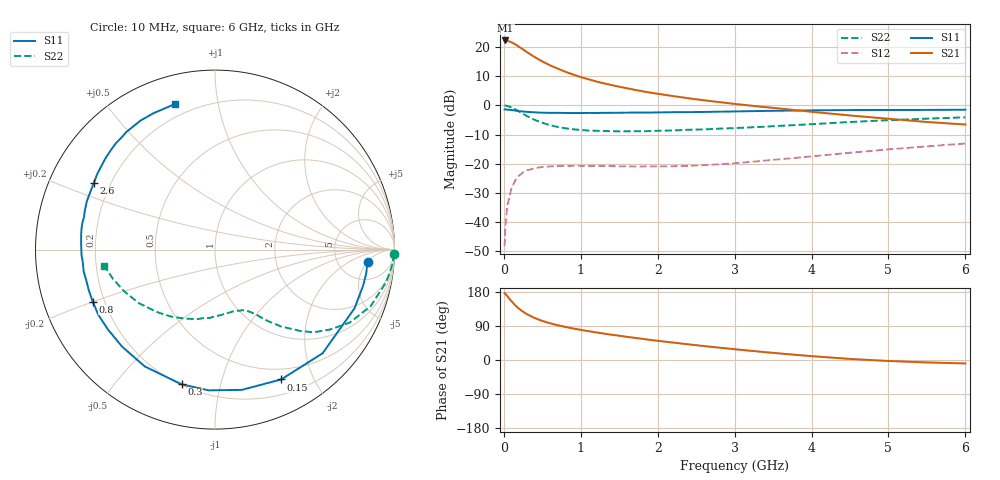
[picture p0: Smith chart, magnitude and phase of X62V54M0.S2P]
! SIEMENS Small Signal Semiconductors
! BFP193W
! Si NPN RF Bipolar Junction Transistor in SOT343
! VCE = 2.5 V  IC = 4 mA
! Common Emitter S-Parameters:  April 1994
# GHz  S  MA  R  50
!  f  S11  S21  S12  S22
! GHz  MAG  ANG  MAG  ANG  MAG  ANG  MAG  ANG
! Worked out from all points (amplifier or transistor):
!   40 points, 10 MHz to 6 GHz, reference 50 ohm
!   highest |S21| = 22.2 dB at 20 MHz (marker M1)
!   |S21| within 3 dB of that: start of sweep to 245.4 MHz
!   unconditionally stable (mu >= 1): 1.781 GHz to 4.478 GHz
!   at 200 MHz: K = 0.12, MSG = 22.0 dB, |S12| = -24.0 dB
!   at 1.5 GHz: K = 0.86, MSG = 13.6 dB, |S12| = -20.9 dB
!   at 6 GHz: K = 0.94, MSG = 3.3 dB, |S12| = -13.1 dB
!   S11 on the Smith chart (normalised r, x): 10 MHz: 10, -5; 150 MHz: 0.37, -1.57; 300 MHz: 0.20, -0.76; 800 MHz: 0.16, -0.20; 2.6 GHz: 0.14, +0.25; 6 GHz: 0.14, +0.75
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0.01  0.8525 -4.5  12.82 176.6  0.0039 87.7  0.9977 -1.4
0.02  0.853 -9.2  12.87 174.8  0.0085 84.6  0.9921 -4.4
0.05  0.8434 -22.8  12.68 167.0  0.0204 78.8  0.9718 -10.6
0.1  0.8325 -43.9  11.95 155.0  0.0381 67.3  0.9226 -20.0
0.15  0.8121 -63.0  11.04 144.0  0.0525 58.1  0.854 -28.4
0.2  0.7956 -79.2  9.977 134.9  0.0631 50.4  0.7815 -34.7
0.25  0.785 -92.5  9.031 127.5  0.0712 44.1  0.717 -40.0
0.3  0.7734 -103.9  8.114 121.0  0.0771 39.3  0.6559 -43.7
0.4  0.7595 -121.0  6.705 110.9  0.0842 31.7  0.5648 -49.3
0.5  0.7484 -133.7  5.641 103.1  0.0882 26.9  0.5031 -53.0
0.6  0.7443 -143.2  4.838 96.9  0.0902 23.4  0.4578 -55.8
0.7  0.7446 -150.8  4.252 91.8  0.0915 21.3  0.4263 -57.7
0.8  0.7405 -157.0  3.751 87.3  0.0922 19.4  0.4049 -59.9
1.1  0.7419 -170.4  2.795 76.1  0.0924 16.9  0.3702 -65.6
1.3  0.7441 -177.5  2.378 69.7  0.0916 16.6  0.3633 -69.8
1.6  0.7504 173.6  1.959 61.1  0.0904 18.0  0.3593 -76.1
2.2  0.763 159.5  1.44 46.0  0.0908 24.0  0.3718 -90.0
2.6  0.7704 151.3  1.221 36.8  0.0946 29.5  0.387 -99.6
3.2  0.7947 140.1  0.992 24.5  0.1075 36.5  0.4196 -113.8
4.5  0.8298 120.1  0.671 2.8  0.1543 41.5  0.5188 -144.9
5.5  0.8345 110.2  0.519 -6.4  0.1987 38.6  0.5919 -164.1
6  0.8413 105.4  0.47 -9.1  0.2223 36.3  0.6237 -171.8
